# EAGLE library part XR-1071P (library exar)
AUDIO PROCESSOR
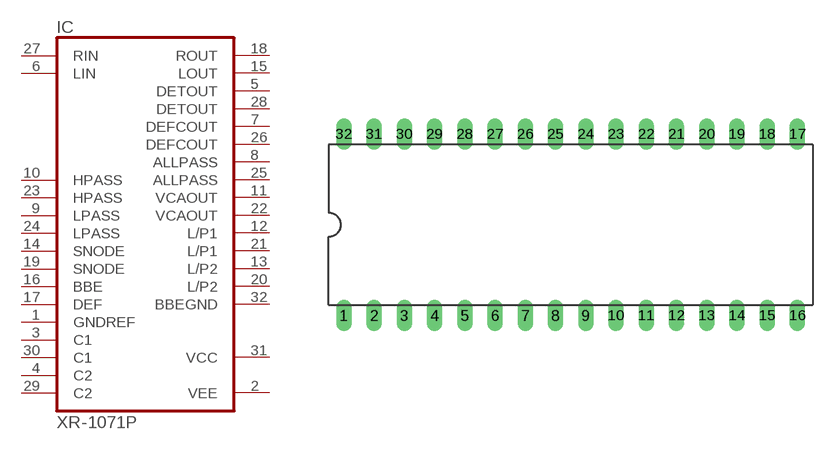
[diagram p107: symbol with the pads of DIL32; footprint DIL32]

Designator prefix IC

## XR-1071P (OC_FARNELL: unknown; OC_NEWARK: unknown)  [DIL32]
1  GNDREF  in
2  VEE  pwr
3  C1  in
4  C2  in
5  DETOUT  out
6  LIN  in
7  DEFCOUT  out
8  ALLPASS  out
9  LPASS  in
10  HPASS  in
11  VCAOUT  out
12  L/P1  out
13  L/P2  out
14  SNODE  in
15  LOUT  out
16  BBE  in
17  DEF  in
18  ROUT  out
19  SNODE  in
20  L/P2  out
21  L/P1  out
22  VCAOUT  out
23  HPASS  in
24  LPASS  in
25  ALLPASS  out
26  DEFCOUT  out
27  RIN  in
28  DETOUT  out
29  C2  in
30  C1  in
31  VCC  pwr
32  BBEGND  out

## Footprint DIL32 (pad centres in mm)
Dual In Line Package
drill 0.813 long: 1 -19.05,-7.62; 2 -16.51,-7.62; 3 -13.97,-7.62; 4 -11.43,-7.62; 5 -8.89,-7.62; 6 -6.35,-7.62; 7 -3.81,-7.62; 8 -1.27,-7.62; 9 1.27,-7.62; 10 3.81,-7.62; 11 6.35,-7.62; 12 8.89,-7.62; 13 11.43,-7.62; 14 13.97,-7.62; 15 16.51,-7.62; 16 19.05,-7.62; 17 19.05,7.62; 18 16.51,7.62; 19 13.97,7.62; 20 11.43,7.62; 21 8.89,7.62; 22 6.35,7.62; 23 3.81,7.62; 24 1.27,7.62; 25 -1.27,7.62; 26 -3.81,7.62; 27 -6.35,7.62; 28 -8.89,7.62; 29 -11.43,7.62; 30 -13.97,7.62; 31 -16.51,7.62; 32 -19.05,7.62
